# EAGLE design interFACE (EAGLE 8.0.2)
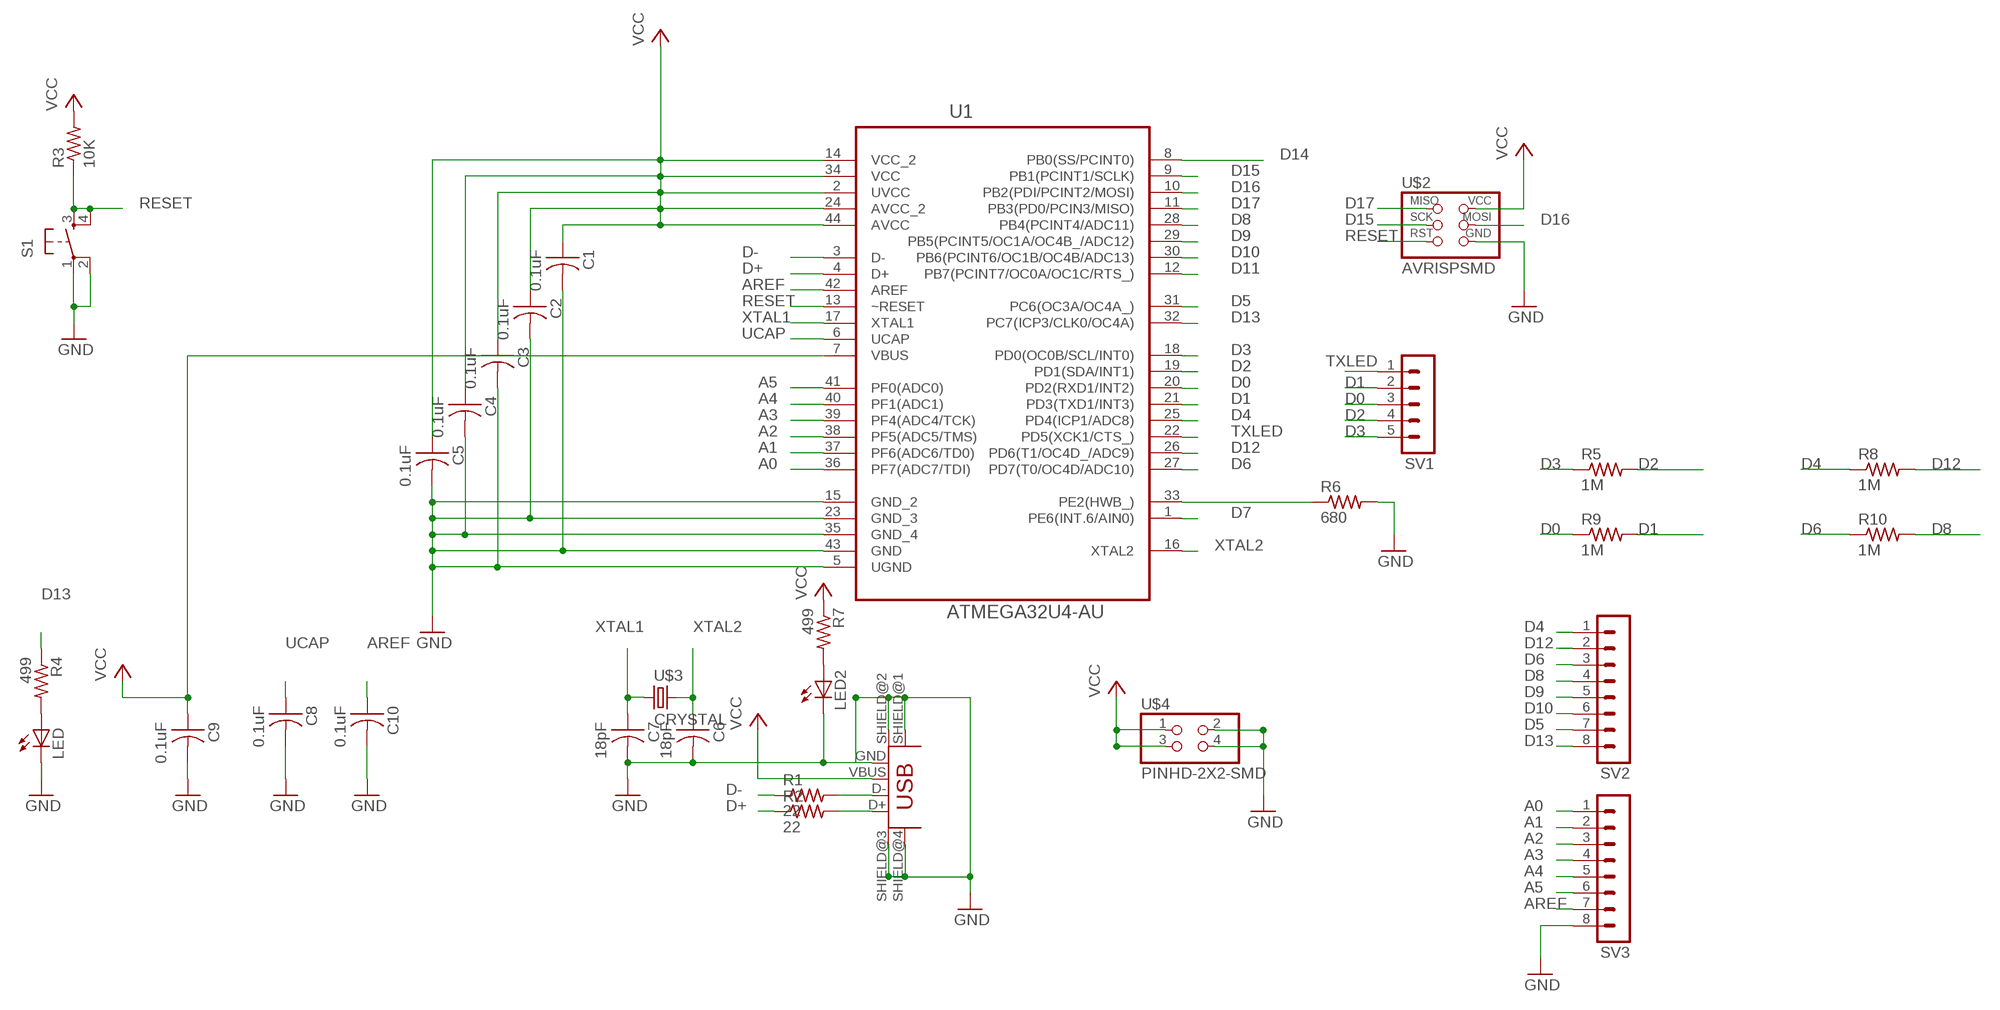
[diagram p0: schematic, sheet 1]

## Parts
C1  0.1uF  CAP-US1206FAB  [C1206FAB]
C2  0.1uF  CAP-US1206FAB  [C1206FAB]
C3  0.1uF  CAP-US1206FAB  [C1206FAB]
C4  0.1uF  CAP-US1206FAB  [C1206FAB]
C5  0.1uF  CAP-US1206FAB  [C1206FAB]
C6  18pF  CAP-US1206FAB  [C1206FAB]
C7  18pF  CAP-US1206FAB  [C1206FAB]
C8  0.1uF  CAP-US1206FAB  [C1206FAB]
C9  0.1uF  CAP-US1206FAB  [C1206FAB]
C10  0.1uF  CAP-US1206FAB  [C1206FAB]
LED  LED1206  [1206]
LED2  LED1206  [1206]
R1  22  RES-US1206FAB  [R1206FAB]
R2  22  RES-US1206FAB  [R1206FAB]
R3  10K  RES-US1206FAB  [R1206FAB]
R4  499  RESISTOR1206  [1206]
R5  1M  RES-US1206FAB  [R1206FAB]
R6  680  RES-US1206FAB  [R1206FAB]
R7  499  RESISTOR1206  [1206]
R8  1M  RES-US1206FAB  [R1206FAB]
R9  1M  RES-US1206FAB  [R1206FAB]
R10  1M  RES-US1206FAB  [R1206FAB]
S1  6MM_SWITCH6MM_SWITCH  [6MM_SWITCH]
SV1  MA05-1  [MA05-1]
SV2  MA08-1  [MA08-1]
SV3  MA08-1  [MA08-1]
U1  ATMEGA32U4-AU  [QFP80P1200X1200X120-44N]
U$1  USB_MINIB  [USB_MINIB]
U$2  AVRISPSMD  [2X03SMD]
U$3  CRYSTAL  [2-SMD-5X3MM]
U$4  PINHD-2X2-SMD  [2X02SMD]

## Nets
A0: SV3.1 U1.36(PF7(ADC7/TDI))
A1: SV3.2 U1.37(PF6(ADC6/TD0))
A2: SV3.3 U1.38(PF5(ADC5/TMS))
A3: SV3.4 U1.39(PF4(ADC4/TCK))
A4: SV3.5 U1.40(PF1(ADC1))
A5: SV3.6 U1.41(PF0(ADC0))
AREF: C10.1 SV3.7 U1.42(AREF)
D0: R9.1 SV1.3 U1.20(PD2(RXD1/INT2))
D1: R9.2 SV1.2 U1.21(PD3(TXD1/INT3))
D2: R5.2 SV1.4 U1.19(PD1(SDA/INT1))
D3: R5.1 SV1.5 U1.18(PD0(OC0B/SCL/INT0))
D4: R8.1 SV2.1 U1.25(PD4(ICP1/ADC8))
D5: SV2.7 U1.31(PC6(OC3A/OC4A_))
D6: R10.1 SV2.3 U1.27(PD7(T0/OC4D/ADC10))
D7: U1.1(PE6(INT.6/AIN0))
D8: R10.2 SV2.4 U1.28(PB4(PCINT4/ADC11))
D9: SV2.5 U1.29(PB5(PCINT5/OC1A/OC4B_/ADC12))
D10: SV2.6 U1.30(PB6(PCINT6/OC1B/OC4B/ADC13))
D11: U1.12(PB7(PCINT7/OC0A/OC1C/RTS_))
D12: R8.2 SV2.2 U1.26(PD6(T1/OC4D_/ADC9))
D13: R4.1 SV2.8 U1.32(PC7(ICP3/CLK0/OC4A))
D14: U1.8(PB0(SS/PCINT0))
D15: U1.9(PB1(PCINT1/SCLK)) U$2.3(SCK)
D16: U1.10(PB2(PDI/PCINT2/MOSI)) U$2.4(MOSI)
D17: U1.11(PB3(PD0/PCIN3/MISO)) U$2.1(MISO)
D+: R2.1 U1.4(D+)
D-: R1.1 U1.3(D-)
GND: C1.2 C2.2 C3.2 C4.2 C5.2 C6.2 C7.2 C8.2 C9.2 C10.2 LED2.2(C) LED.2(C) R6.2 S1.1(P) S1.2(P1) SV3.8 U1.5(UGND) U1.15(GND_2) U1.23(GND_3) U1.35(GND_4) U1.43(GND) U$1.GND U$1.SHIELD@1(SHIELD) U$1.SHIELD@2(SHIELD1) U$1.SHIELD@3(SHIELD2) U$1.SHIELD@4(SHIELD3) U$2.6(GND) U$4.2 U$4.4
N$1: R1.2 U$1.D-
N$2: R2.2 U$1.D+
N$3: LED.1(A) R4.2
N$5: LED2.1(A) R7.2
N$35: R6.1 U1.33(PE2(HWB_))
RESET: R3.1 S1.3(S) S1.4(S1) U1.13(~RESET) U$2.5(RST)
TXLED: SV1.1 U1.22(PD5(XCK1/CTS_))
UCAP: C8.1 U1.6(UCAP)
VCC: C1.1 C2.1 C3.1 C4.1 C5.1 C9.1 R3.2 R7.1 U1.2(UVCC) U1.7(VBUS) U1.14(VCC_2) U1.24(AVCC_2) U1.34(VCC) U1.44(AVCC) U$1.VBUS U$2.2(VCC) U$4.1 U$4.3
XTAL1: C7.1 U1.17(XTAL1) U$3.P$1
XTAL2: C6.1 U1.16(XTAL2) U$3.P$2

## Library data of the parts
C1-C10 = fab:CAP-US
LED LED2 = ng:LED
R1-R3 R5 R6 R8-R10 = fab:RES-US: Resistor (US Symbol)
R4 R7 = ng:RESISTOR
S1 = ng:6MM_SWITCH: OMRON SWITCH
SV1 = con-lstb:MA05-1: PIN HEADER; OC_FARNELL: unknown; OC_NEWARK: unknown
SV2 SV3 = con-lstb:MA08-1: PIN HEADER
U1 = Atmel_By_element14_Batch_1:ATMEGA32U4-AU: 8-bit Microcontroller with ISP Flash and USB Controller; MPN: ATMEGA32U4-AU; OC_FARNELL: 1748525; OC_NEWARK: 26R5633; PACKAGE: TQFP-44; SUPPLIER: Atmel
U$1 = fab:USB_MINIB
U$2 = fab:AVRISP
U$3 = fab:CRYSTAL
U$4 = fab:PINHD-2X2-SMD

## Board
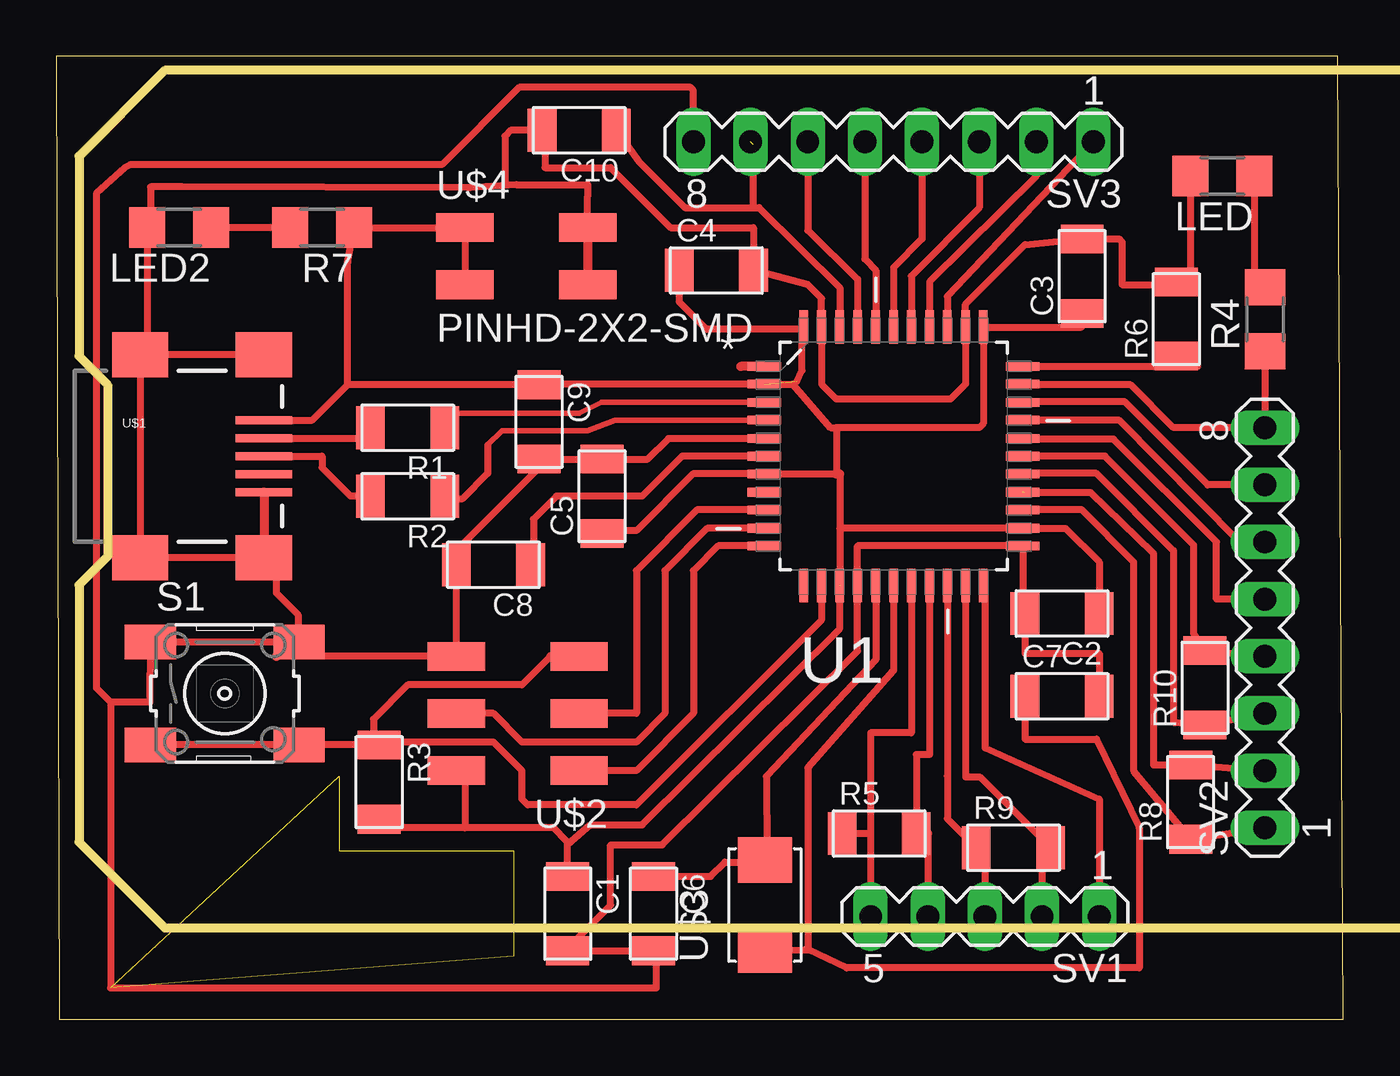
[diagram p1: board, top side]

Size 57.2 x 42.79 mm. Coordinates in mm from the lower left corner, seen from the top.
Outline: 0.13,0 57.2,0 56.95,42.79 0,42.79 0.13,0
Copper layers (1*16): Top 0.035mm / dielectric 1.5mm / Bottom 0.035mm
Design rules "default *": minimum track width 10mil, minimum drill 24mil, track to track 0.4mm, track to pad 0.4mm, pad to pad 0.4mm, via to via 0.4mm, smd to smd 0.4mm, copper to edge 40mil, drill to drill 0.4mm, minimum pad ring 10mil, minimum via ring 8mil, stop-mask expansion 4mil, vias tented up to drill 0mil, thermal gap 10mil
Milling: area 1,4.1 to 101.3,42.2

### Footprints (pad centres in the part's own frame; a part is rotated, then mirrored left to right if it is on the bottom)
C1206FAB = smd 1.27 x 1.905: 1 -1.651,0; 2 1.651,0
1206 = smd 1.6 x 1.803: 1 -1.422,0; 2 1.422,0
R1206FAB = smd 1.27 x 1.905: 1 -1.651,0; 2 1.651,0
6MM_SWITCH = smd 2.286 x 1.524: 1 -3.302,2.286; 2 3.302,2.286; 3 -3.302,-2.286; 4 3.302,-2.286
MA05-1 = drill 1.016 long: 1 -5.08,0; 2 -2.54,0; 3 0,0; 4 2.54,0; 5 5.08,0
MA08-1 = drill 1.016 long: 1 -8.89,0; 2 -6.35,0; 3 -3.81,0; 4 -1.27,0; 5 1.27,0; 6 3.81,0; 7 6.35,0; 8 8.89,0
QFP80P1200X1200X120-44N = smd 1.5 x 0.38: 1 -5.74,3.988; 2 -5.74,3.2; 3 -5.74,2.388; 4 -5.74,1.6; 5 -5.74,0.787; 6 -5.74,0; 7 -5.74,-0.787; 8 -5.74,-1.6; 9 -5.74,-2.388; 10 -5.74,-3.2; 11 -5.74,-3.988; 23 5.74,-3.988; 24 5.74,-3.2; 25 5.74,-2.388; 26 5.74,-1.6; 27 5.74,-0.787; 28 5.74,0; 29 5.74,0.787; 30 5.74,1.6; 31 5.74,2.388; 32 5.74,3.2; 33 5.74,3.988 | smd 0.38 x 1.5: 12 -3.988,-5.74; 13 -3.2,-5.74; 14 -2.388,-5.74; 15 -1.6,-5.74; 16 -0.787,-5.74; 17 0,-5.74; 18 0.787,-5.74; 19 1.6,-5.74; 20 2.388,-5.74; 21 3.2,-5.74; 22 3.988,-5.74; 34 3.988,5.74; 35 3.2,5.74; 36 2.388,5.74; 37 1.6,5.74; 38 0.787,5.74; 39 0,5.74; 40 -0.787,5.74; 41 -1.6,5.74; 42 -2.388,5.74; 43 -3.2,5.74; 44 -3.988,5.74
USB_MINIB = smd 2.5 x 0.35: D+ 3.77,0; D- 3.77,0.8; GND 3.77,-1.6; ID 3.77,-0.8; VBUS 3.77,1.6 | smd 2.5 x 2: SHIELD@1 -1.73,-4.5; SHIELD@2 -1.73,4.5; SHIELD@3 3.77,4.5; SHIELD@4 3.77,-4.5
2X03SMD = smd 2.54 x 1.27: 1 -2.54,2.54; 2 2.92,2.54; 3 -2.54,0; 4 2.92,0; 5 -2.54,-2.54; 6 2.92,-2.54
2-SMD-5X3MM = smd 2 x 2.4: P$1 -2,0; P$2 2,0
2X02SMD = smd 2.54 x 1.27: 1 -2.54,1.27; 2 2.92,1.27; 3 -2.54,-1.27; 4 2.92,-1.27

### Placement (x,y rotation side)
C1  22.73,4.7 270 top
C2  44.7,18.03 180 top
C3  45.59,33.02 90 top
C4  29.34,33.27 0 top
C5  24.26,23.24 90 top
C6  26.54,4.7 270 top
C7  44.7,14.35 0 top
C8  19.43,20.19 180 top
C9  21.46,26.54 270 top
C10  23.24,39.5 180 top
LED  51.82,37.46 180 top
LED2  5.46,35.18 180 top
R1  15.62,26.29 180 top
R2  15.62,23.24 180 top
R3  14.35,10.54 270 top
R4  53.72,31.12 90 top
R5  36.58,8.25 0 top
R6  49.78,31.12 90 top
R7  11.81,35.18 180 top
R8  50.42,9.65 90 top
R9  42.55,7.62 0 top
R10  51.05,14.73 90 top
S1  7.49,14.48 0 top
SV1  41.28,4.57 180 top
SV2  53.72,17.4 90 top
SV3  37.21,38.99 180 top
U1  37.21,25.02 0 top
U$1  5.46,25.02 0 top
U$2  20.7,13.59 180 top
U$3  31.5,5.08 90 top
U$4  20.7,33.91 0 top

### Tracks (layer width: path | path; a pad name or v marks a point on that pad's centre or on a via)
A0
  Top 0.305: SV3.1 39.6,32.12 U1.36
A1
  Top 0.305: SV3.2 43.56,37.46 38.81,32.77 U1.37
A2
  Top 0.305: SV3.3 41.02,36.07 38,33.02 U1.38
A3
  Top 0.305: SV3.4 38.48,34.67 37.21,33.4 U1.39
A4
  Top 0.305: SV3.5 35.94,33.78 36.42,33.27 U1.40
A5
  Top 0.305: SV3.6 33.4,35.05 35.61,32.89 U1.41
AREF  (1 unrouted)
  Top 0.305: C10.1 25.91,38.1 27.94,36.07 30.99,36.07 | 30.99,36.07 30.99,38.86 | 30.99,36.07 31.24,36.07 34.82,32.51 U1.42
D0
  Top 0.305: U1.20 39.6,10.82 39.6,8.91 R9.1 | 41.28,7.62 SV1.3
  Top 0.406: R9.1 41.28,7.62
D1
  Top 0.305: U1.21 40.41,10.77 41.05,10.77 R9.2 | 43.82,7.62 SV1.2
  Top 0.406: R9.2 43.82,7.62
D2
  Top 0.305: U1.19 38.81,11.76 38.23,11.76 R5.2 | 38.74,8.25 SV1.4
  Top 0.406: R5.2 38.74,8.25
D3
  Top 0.305: U1.18 38,12.72 36.2,12.72 36.2,8.25 | 36.2,8.25 R5.1 | 36.2,8.25 SV1.5
D4
  Top 0.305: U1.25 45.59,22.63 47.88,20.32 47.88,11.05 R8.1 SV2.1
D5
  Top 0.305: SV2.7 51.18,23.75 47.5,27.43 42.98,27.43 U1.31
D6
  Top 0.305: U1.27 42.98,24.26 46.23,24.26 49.66,20.83 49.66,13.21 R10.1 SV2.3
D7
  Top 0.406: U1.1 30.43,29.01
D8
  Top 0.305: U1.28 46.61,25.02 50.55,21.08 50.55,17.14 R10.2 SV2.4
D9
  Top 0.305: SV2.5 51.56,18.67 51.56,21.21 46.99,25.78 42.98,25.78 U1.29
D10
  Top 0.305: SV2.6 52.58,21.21 47.24,26.61 43.03,26.61 U1.30
D12  (1 unrouted)
  Top 0.305: 43.03,23.41 45.97,23.41 48.77,20.7 48.77,11.3 R8.2 SV2.2
D13
  Top 0.305: U1.32 42.98,28.19 47.75,28.19 49.66,26.29 SV2.8 R4.1
D15
  Top 0.305: U1.9 28.47,22.63 25.78,19.94 25.78,13.59 U$2.3
D16
  Top 0.305: U1.10 28.93,21.82 27.05,19.94 27.05,13.59 25.78,12.32 20.7,12.32 19.43,13.59 U$2.4
D17
  Top 0.305: U1.11 29.41,21.03 28.32,19.94 28.32,13.59 25.78,11.05 U$2.1
D+
  Top 0.254: U1.4 24.84,26.62 23.62,26.16 19.81,26.16 19.18,25.53
  Top 0.305: 19.18,25.53 19.18,24.26 18.03,23.11 17.4,23.11 R2.1
D-
  Top 0.254: U1.3 24.23,27.41 23.24,26.92 17.4,26.92
  Top 0.305: 17.4,26.92 17.14,26.42 R1.1
GND  (5 unrouted)
  Top 0.305: U$1.SHIELD@4 U$1.SHIELD@1 U$1.SHIELD@2 U$1.SHIELD@3 | U1.5 27.2,25.81 26.29,24.89 C5.2 C9.2 | LED2.2 4.04,29.83 | U$2.6 9.78,16.13 | C8.2 U$2.6 | 4.19,35.33 4.19,36.98 5.59,36.99 18.29,36.96 | U$4.4 23.62,36.58 23.62,37.08 20.45,37.08 19.81,37.05 | 21.46,24.51 18.16,21.21 18.16,20.57 | 18.41,36.96 18.29,36.96 | 19.81,37.05 18.29,36.96 | 2.41,14.1 4.17,14.08 S1.1 S1.2 10.74,16.82 10.74,17.98 9.78,18.95 9.78,19.97 | 2.41,14.1 2.41,1.4 26.67,1.4 26.67,3.56 C6.2 25.84,3.15 26.45,3.05 C1.2 22.99,3.43 24.64,5.08 24.64,7.75 26.92,7.75 35.61,16.36 35.61,21.03 U1.23 42.95,18.14 C2.2 43.05,16.26 46.36,16.26 C7.2 | LED.2 50.39,32.77 R6.2 49.66,32.64 47.37,32.64 47.37,34.54 47.24,34.67 C3.2 43.05,34.42 40.41,31.78 U1.35 40.41,28.22 39.75,27.56 34.67,27.56 34.01,28.22 U1.43 34.01,32.03 33.4,32.64 C4.2 30.99,35.18 27.3,35.18 24.64,37.85 21.72,37.85 21.72,39.37 C10.2 20.19,39.5 19.94,39.24 19.94,37.17 19.81,37.05 | 2.41,14.1 1.78,14.73 1.78,36.7 3.05,37.85 3.3,37.97 17.14,37.97 20.57,41.4 28.19,41.4 28.32,41.27 SV3.8
  Top 0.406: U$1.GND U$1.SHIELD@4 9.78,19.97 | U$1.SHIELD@3 9.27,29.52 | 4.04,29.83 U$1.SHIELD@2 | 9.78,16.13 S1.2 | U$4.2 U$4.4 | C9.2 21.46,24.51 | 18.16,20.57 C8.2 | U$2.6 | 4.19,35.33 LED2.2
N$1
  Top 0.305: U$1.D- 13.97,25.82
  Top 0.406: 13.97,25.82 R1.2
N$2
  Top 0.305: R2.2 13.08,23.24 11.81,24.51 11.81,25.02 U$1.D+
N$3
  Top 0.305: LED.1 53.24,32.54 R4.2
N$5
  Top 0.305: R7.2 LED2.1
N$35
  Top 0.305: U1.33 50.72,29.01 R6.1
RESET
  Top 0.305: S1.4 S1.3 | 21.97,16.13 20.7,14.86 15.62,14.86 14.1,13.33 14.1,12.45 R3.1 9.78,12.19 | 14.48,12.32 19.43,12.32 20.7,11.05 20.7,9.78 20.95,9.53 25.78,9.53 34.02,17.76 34.02,19.25 U1.13
  Top 0.406: 14.48,12.32 R3.1 | U$2.5 21.97,16.13 | 9.78,12.19 S1.4
TXLED
  Top 0.305: U1.22 41.28,19.28 41.28,12.06 46.36,9.78 SV1.1
UCAP
  Top 0.305: U1.6 27.81,25.02 26.04,23.24 22.22,23.24 21.21,22.23 21.21,20.32 C8.1
VCC  (2 unrouted)
  Top 0.305: 32.92,28.35 33.15,28.83 33.15,30.68 | 21.49,28.22 U1.2 32.74,28.22 34.42,26.29 34.67,26.29 | C9.1 12.95,28.19 | 12.95,28.19 11.38,26.62 U$1.VBUS | 12.95,28.19 12.95,33.63 R7.1 U$4.1 U$4.3 | C3.1 45.57,30.76 U1.34 41.2,26.47 41.02,26.29 34.67,26.29 | 33.22,30.66 28.91,30.66 27.69,31.88 C4.1 | 18.16,8.51 14.73,8.51 R3.2 | 18.16,11.05 18.16,8.51 | 18.16,8.51 22.1,8.51 22.73,7.87 C1.1 22.73,7.75 23.75,8.64 26.04,8.64 34.82,17.36 U1.14 | 34.82,24.23 34.82,21.82 | 34.82,21.82 U1.14 | 34.82,21.82 U1.24 44.86,21.82 46.36,20.32 C2.1 | 34.67,26.29 34.67,24.23 U1.7 28.3,24.23 25.78,21.72 23.88,21.72 C5.1
  Top 0.406: 33.15,30.68 U1.44 33.22,30.66 | 41.28,30.68 U1.34 | 21.49,28.22 C9.1 | U$2.2 18.16,11.05 | 34.67,24.23 34.82,24.23
XTAL1
  Top 0.305: U$3.P$1 33.28,3.08 | 33.28,3.08 33.44,3.08 35.12,2.29 48.13,2.29 48.13,8.51 46.23,12.45 43.05,12.45 C7.1 | U1.17 37.21,15.49 33.4,11.18 33.4,3.21 33.28,3.08
XTAL2
  Top 0.305: U1.16 36.42,15.98 31.56,10.79 31.59,7.37 U$3.P$2 31.4,6.98 29.72,6.98 29.08,6.35 C6.1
